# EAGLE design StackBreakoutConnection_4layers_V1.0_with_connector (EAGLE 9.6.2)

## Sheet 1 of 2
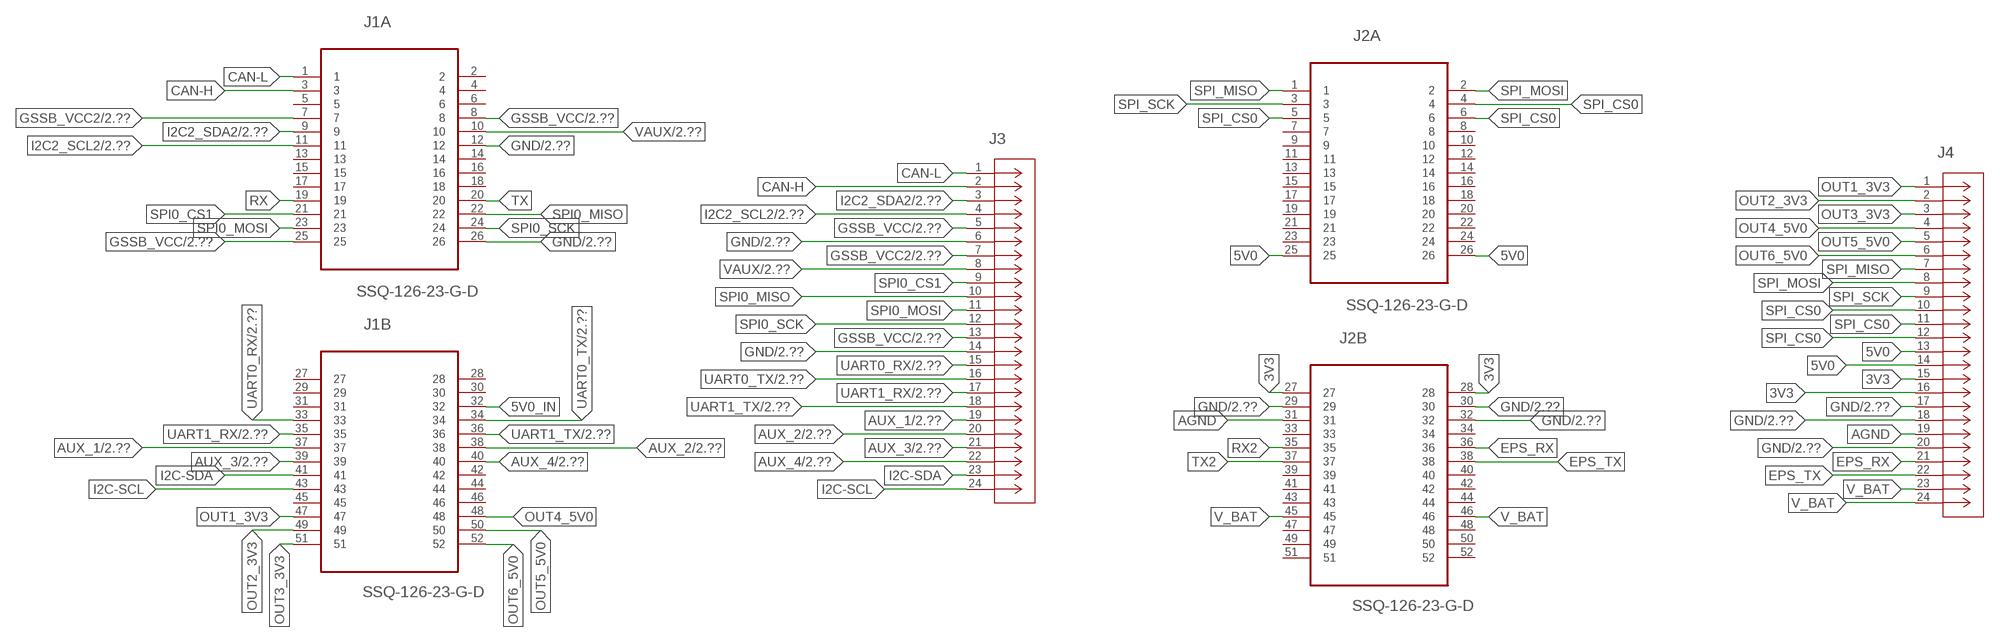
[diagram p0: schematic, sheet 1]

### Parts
J1  SSQ-126-23-G-D  [SAMTEC_SSQ-126-23-G-D]
J2  SSQ-126-23-G-D  [SAMTEC_SSQ-126-23-G-D]
J3  2086592440  [CON_2086592440_MOL]
J4  2086592440  [CON_2086592440_MOL]

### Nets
3V3: J2.27 J2.28 J4.15 J4.16
5V0: J2.25 J2.26 J4.13 J4.14
5V0_IN: J1.32
AGND: J2.31 J4.19
AUX_1: J1.37 J3.19 ; also sheet 2
AUX_2: J1.38 J3.20 ; also sheet 2
AUX_3: J1.39 J3.21 ; also sheet 2
AUX_4: J1.40 J3.22 ; also sheet 2
CAN-H: J1.3 J3.2
CAN-L: J1.1 J3.1
EPS_RX: J2.36 J4.21
EPS_TX: J2.38 J4.22
GND: J1.12 J1.26 J2.29 J2.30 J2.32 J3.6 J3.14 J4.17 J4.18 J4.20 ; also sheet 2
GSSB_VCC: J1.8 J1.25 J3.5 J3.13 ; also sheet 2
GSSB_VCC2: J1.7 J3.7 ; also sheet 2
I2C2_SCL2: J1.11 J3.4 ; also sheet 2
I2C2_SDA2: J1.9 J3.3 ; also sheet 2
I2C-SCL: J1.43 J3.24
I2C-SDA: J1.41 J3.23
OUT1_3V3: J1.47 J4.1
OUT2_3V3: J1.49 J4.2
OUT3_3V3: J1.51 J4.3
OUT4_5V0: J1.48 J4.4
OUT5_5V0: J1.50 J4.5
OUT6_5V0: J1.52 J4.6
RX: J1.19
RX2: J2.35
SPI0_CS1: J1.21 J3.9
SPI0_MISO: J1.22 J3.10
SPI0_MOSI: J1.23 J3.11
SPI0_SCK: J1.24 J3.12
SPI_CS0: J2.4 J2.5 J2.6 J4.10 J4.11 J4.12
SPI_MISO: J2.1 J4.7
SPI_MOSI: J2.2 J4.8
SPI_SCK: J2.3 J4.9
TX: J1.20
TX2: J2.37
UART0_RX: J1.33 J3.15 ; also sheet 2
UART0_TX: J1.34 J3.16 ; also sheet 2
UART1_RX: J1.35 J3.17 ; also sheet 2
UART1_TX: J1.36 J3.18 ; also sheet 2
V_BAT: J2.45 J2.46 J4.23 J4.24
VAUX: J1.10 J3.8 ; also sheet 2
Unconnected: J1.2 J1.4 J1.5 J1.6 J1.13 J1.14 J1.15 J1.16 J1.17 J1.18 J1.27 J1.28 J1.29 J1.30 J1.31 J1.42 J1.44 J1.45 J1.46 J2.7 J2.8 J2.9 J2.10 J2.11 J2.12 J2.13 J2.14 J2.15 J2.16 J2.17 J2.18 J2.19 J2.20 J2.21 J2.22 J2.23 J2.24 J2.33 J2.34 J2.39 J2.40 J2.41 J2.42 J2.43 J2.44 J2.47 J2.48 J2.49 J2.50 J2.51 J2.52

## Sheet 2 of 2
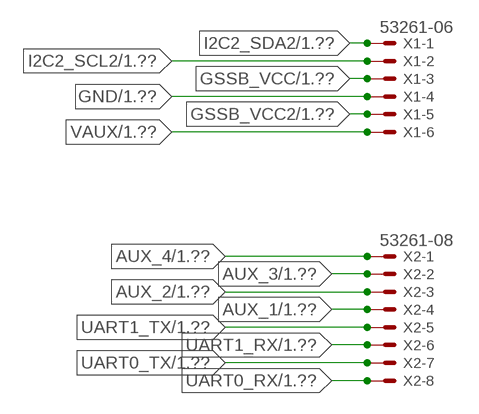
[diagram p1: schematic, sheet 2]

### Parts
X1  53261-06  [53261-06]
X2  53261-08  [53261-08]

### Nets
AUX_1: X2.4 ; also sheet 1
AUX_2: X2.3 ; also sheet 1
AUX_3: X2.2 ; also sheet 1
AUX_4: X2.1 ; also sheet 1
GND: X1.4 ; also sheet 1
GSSB_VCC: X1.3 ; also sheet 1
GSSB_VCC2: X1.5 ; also sheet 1
I2C2_SCL2: X1.2 ; also sheet 1
I2C2_SDA2: X1.1 ; also sheet 1
UART0_RX: X2.8 ; also sheet 1
UART0_TX: X2.7 ; also sheet 1
UART1_RX: X2.6 ; also sheet 1
UART1_TX: X2.5 ; also sheet 1
VAUX: X1.6 ; also sheet 1

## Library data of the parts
J1 J2 = SPEL:SSQ-126-23-G-D: CONN RECEPTACLE, 2.54MM, DUAL, 52WAY; MPN: SSQ-126-23-G-D; OC_FARNELL: -; OC_NEWARK: 82P0504; PACKAGE: RECEPTACLE, 2.54MM, DUAL, 52WAY; SUPPLIER: Samtec
J3 J4 = MolexP24:2086592440; BUILT_BY: Molex_Team; COPYRIGHT: Copyright (C) 2018 Accelerated Designs. All rights reserved; DESCRIPTION: 2.00mm Pitch, iGrid PCB Header, Dual Row, Right-Angle, Through Hole, 0.10µm Gold (Au) Plating, Positive Lock, 24 Circuits, Tray, 3.20mm PC Tail Length, Natural; MANUFACTURER_PART_NUMBER: 2086592440; SOURCELIBRARY: Add_to_database_2021-04-21; VENDOR: Molex Connector Corporation
X1 = con-molex:53?-06: CONNECTOR wire to board 1.25 mm (.049 inch) pitch header; MF: MOLEX; OC_FARNELL: 1125375; OC_NEWARK: unknown
X2 = con-molex:53?-08: CONNECTOR wire to board 1.25 mm (.049 inch) pitch header; MF: MOLEX; OC_FARNELL: 1125376; OC_NEWARK: unknown

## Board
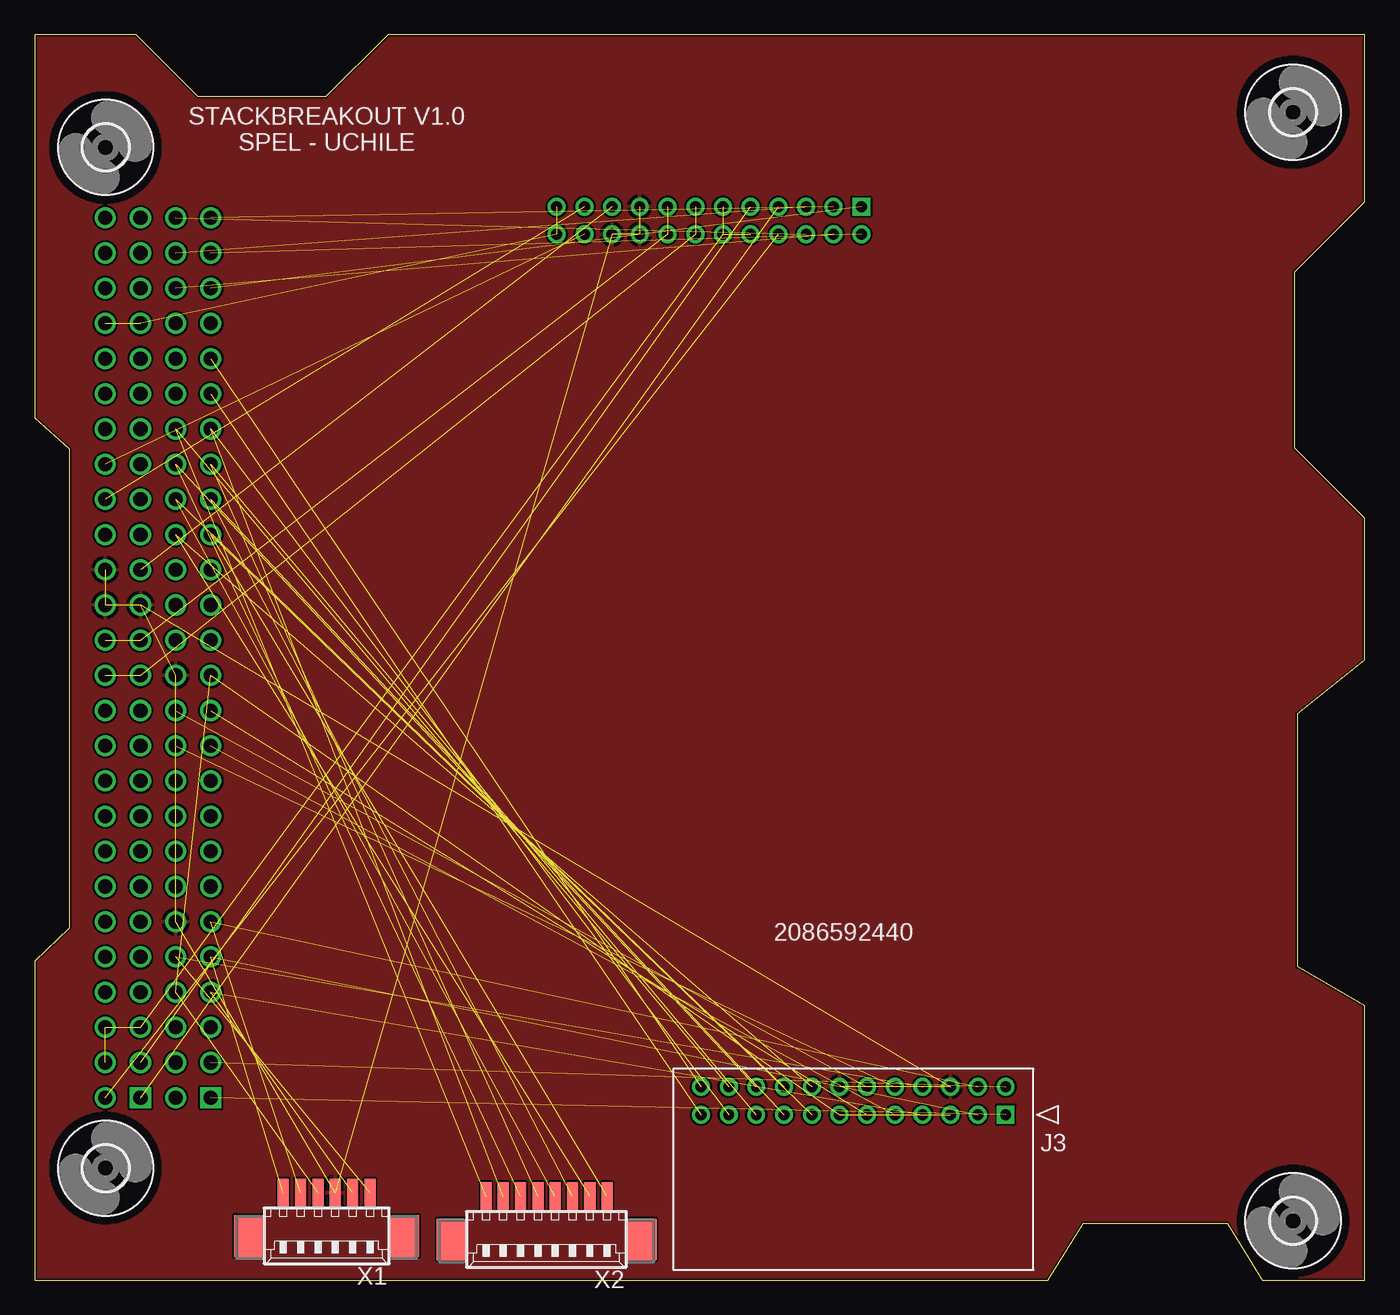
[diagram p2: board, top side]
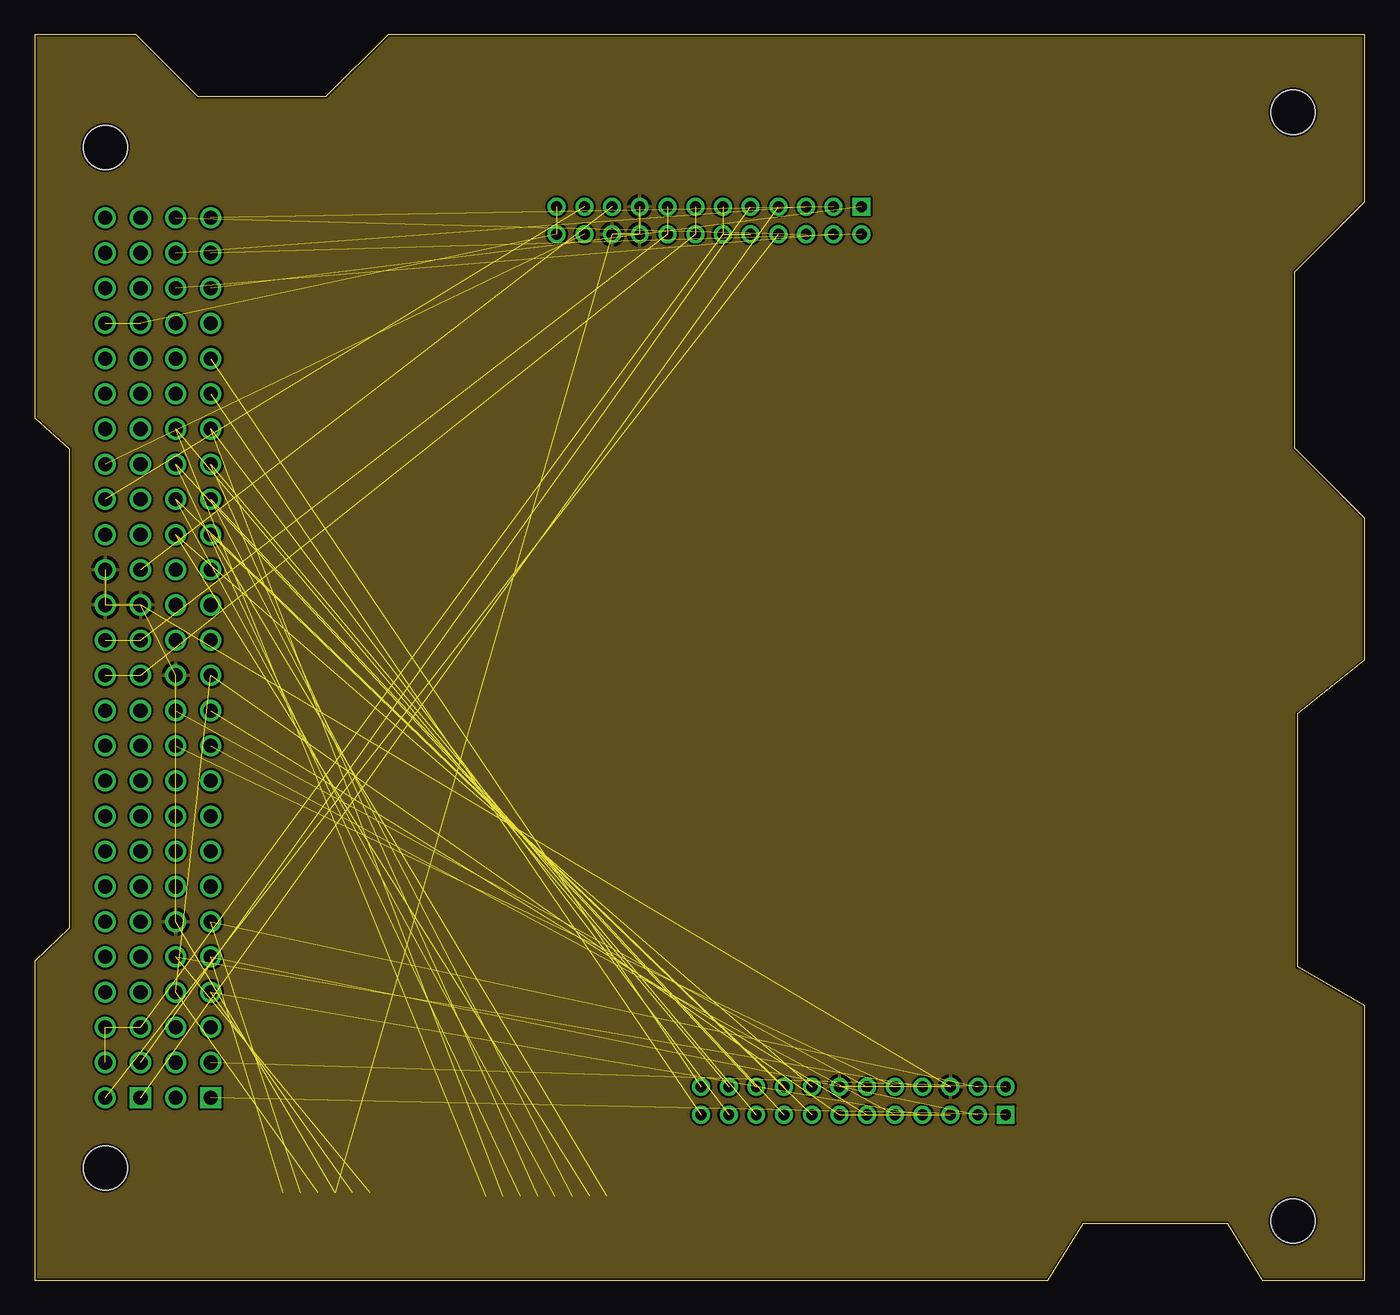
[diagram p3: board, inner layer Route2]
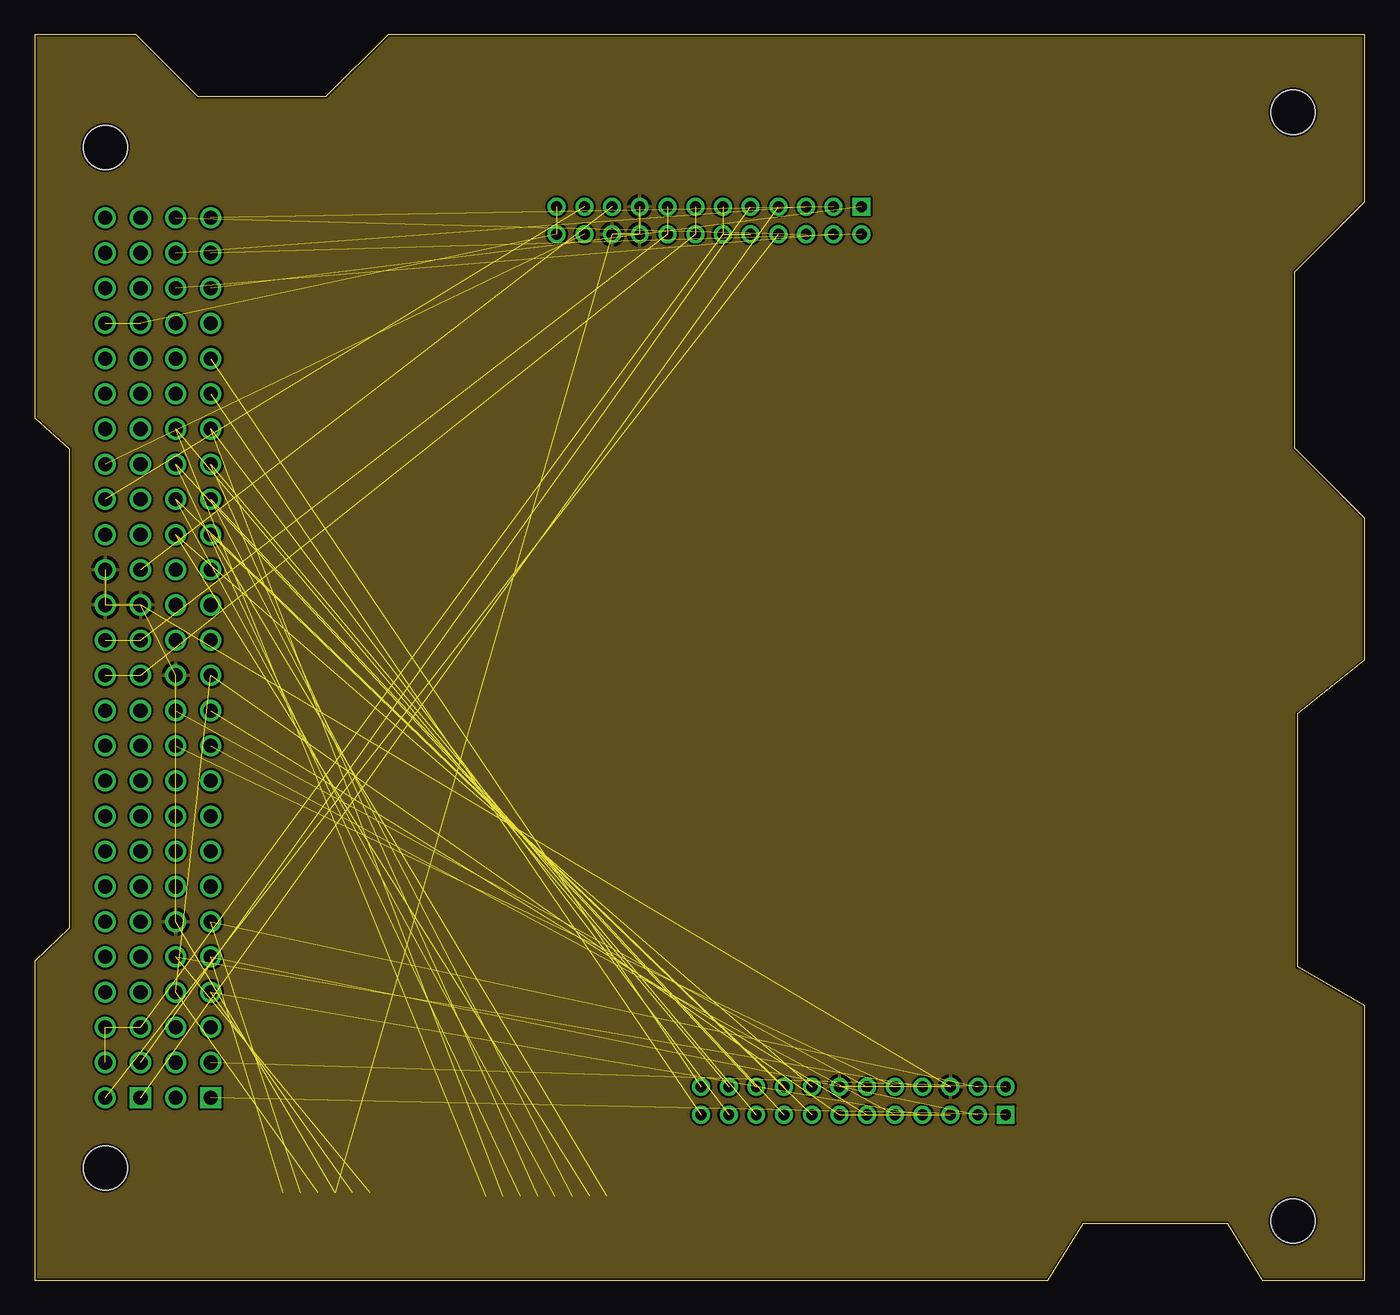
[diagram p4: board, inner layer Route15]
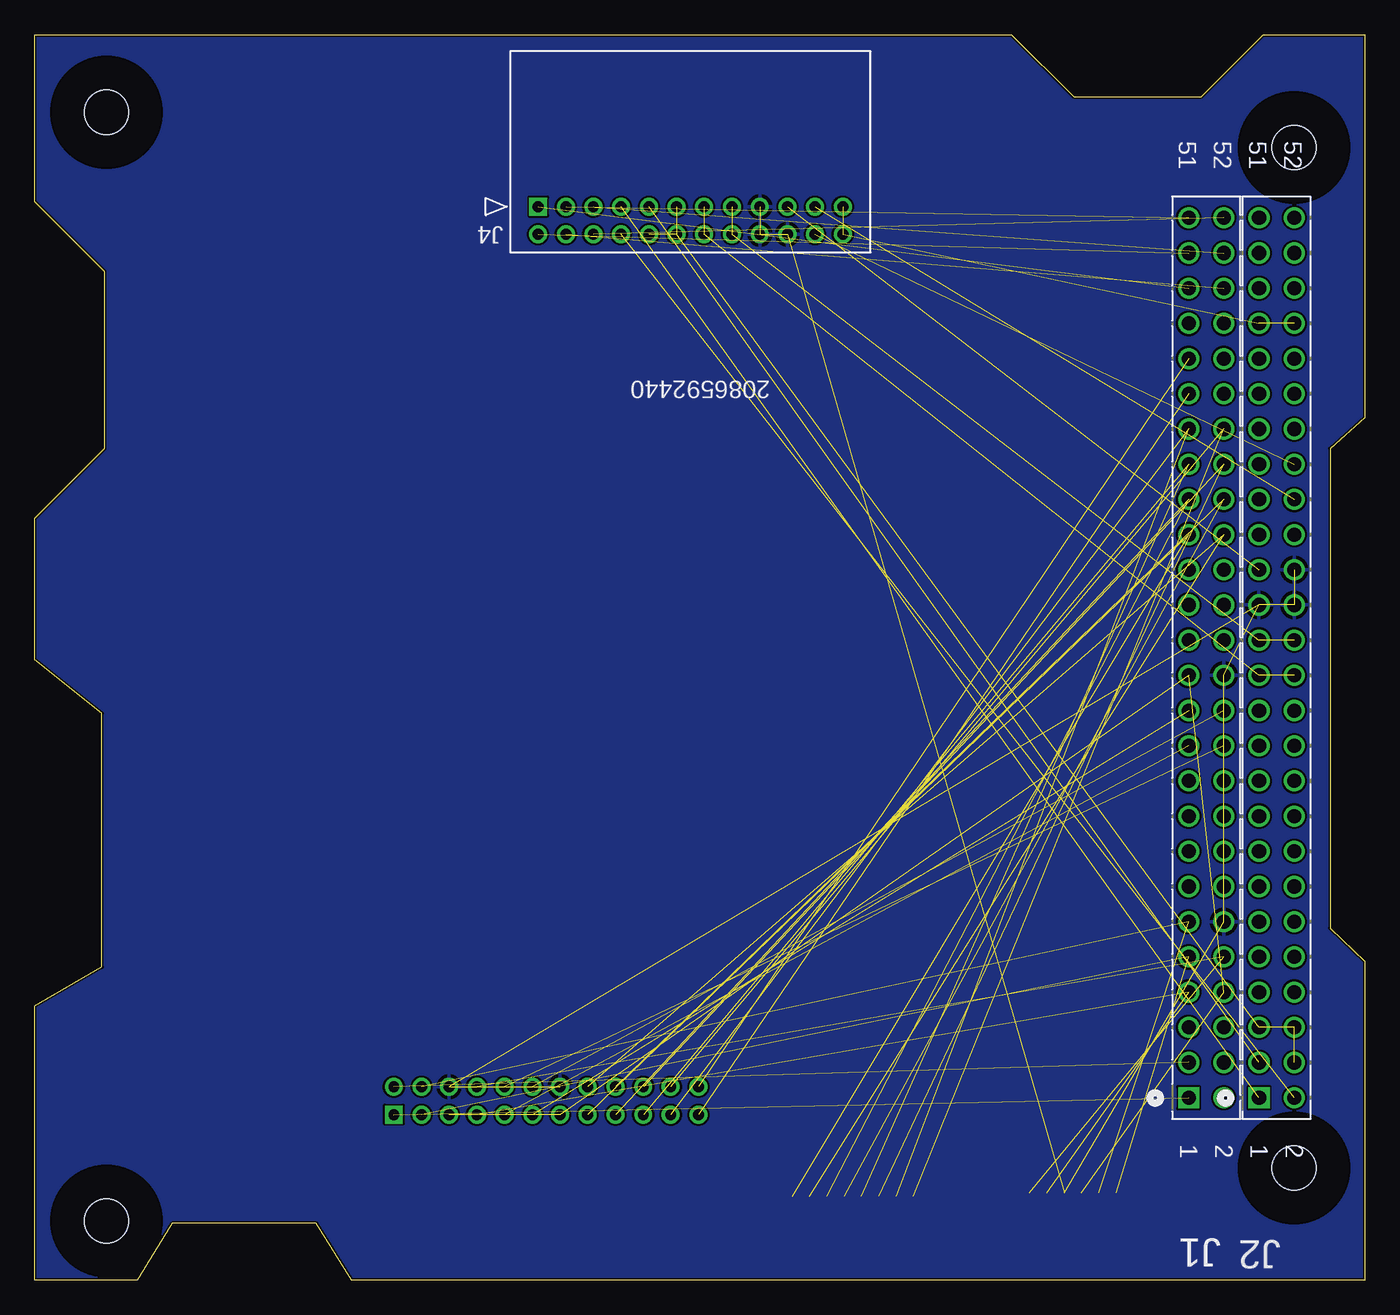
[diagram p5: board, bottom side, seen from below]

Size 96.04 x 89.88 mm. Coordinates in mm from the lower left corner, seen from the top.
Outline: 90.98,72.77 96.04,77.83 96.04,89.88 25.51,89.88 21.02,85.4 11.8,85.4 7.32,89.88 0,89.88 0,62.23 2.5,60 2.5,25.4 0,23 0,0 73.15,0 75.7,4.1 86.09,4.1 88.65,0 96.01,0 96.01,19.81 91.19,22.61 91.19,40.89 96.04,44.76 96.04,54.97 90.98,60.02 90.98,72.77
Copper layers (1+2*15+16): Top 0.035mm / dielectric 1.5mm / Route2 0.035mm / dielectric 0.15mm / Route15 0.035mm / dielectric 0.2mm / Bottom 0.035mm
Design rules "default *": minimum track width 20mil, minimum drill 0.2mm, track to track 6mil, track to pad 6mil, pad to pad 6mil, via to via 6mil, smd to smd 6mil, copper to edge 6mil, drill to drill 6mil, minimum pad ring 10mil, minimum via ring 8mil, stop-mask expansion 4mil, vias tented up to drill 0mil, thermal gap 10mil

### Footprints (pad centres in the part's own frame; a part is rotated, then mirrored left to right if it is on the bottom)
SAMTEC_SSQ-126-23-G-D = drill 1.016 square: 1 63.5,-2.54 | drill 1.016: 2 63.5,0; 3 60.96,-2.54; 4 60.96,0; 5 58.42,-2.54; 6 58.42,0; 7 55.88,-2.54; 8 55.88,0; 9 53.34,-2.54; 10 53.34,0; 11 50.8,-2.54; 12 50.8,0; 13 48.26,-2.54; 14 48.26,0; 15 45.72,-2.54; 16 45.72,0; 17 43.18,-2.54; 18 43.18,0; 19 40.64,-2.54; 20 40.64,0; 21 38.1,-2.54; 22 38.1,0; 23 35.56,-2.54; 24 35.56,0; 25 33.02,-2.54; 26 33.02,0; 27 30.48,-2.54; 28 30.48,0; 29 27.94,-2.54; 30 27.94,0; 31 25.4,-2.54; 32 25.4,0; 33 22.86,-2.54; 34 22.86,0; 35 20.32,-2.54; 36 20.32,0; 37 17.78,-2.54; 38 17.78,0; 39 15.24,-2.54; 40 15.24,0; 41 12.7,-2.54; 42 12.7,0; 43 10.16,-2.54; 44 10.16,0; 45 7.62,-2.54; 46 7.62,0; 47 5.08,-2.54; 48 5.08,0; 49 2.54,-2.54; 50 2.54,0; 51 0,-2.54; 52 0,0
CON_2086592440_MOL = drill 0.787 pad 1.143 square: 1 0,0 | drill 0.787 pad 1.143: 2 0,2.007; 3 -2.007,0; 4 -2.007,2.007; 5 -3.988,0; 6 -3.988,2.007; 7 -5.994,0; 8 -5.994,2.007; 9 -8.001,0; 10 -8.001,2.007; 11 -10.008,0; 12 -10.008,2.007; 13 -11.989,0; 14 -11.989,2.007; 15 -13.995,0; 16 -13.995,2.007; 17 -16.002,0; 18 -16.002,2.007; 19 -18.009,0; 20 -18.009,2.007; 21 -19.99,0; 22 -19.99,2.007; 23 -21.996,0; 24 -21.996,2.007
3,2 = hole 3.2: 0,0
53261-06 = smd 0.8 x 2: 1 3.125,-2.5; 2 1.875,-2.5; 3 0.625,-2.5; 4 -0.625,-2.5; 5 -1.875,-2.5; 6 -3.125,-2.5 | smd 2.1 x 3: S1 5.625,0.625; S2 -5.625,0.625
53261-08 = smd 0.8 x 2: 1 4.375,-2.5; 2 3.125,-2.5; 3 1.875,-2.5; 4 0.625,-2.5; 5 -0.625,-2.5; 6 -1.875,-2.5; 7 -3.125,-2.5; 8 -4.375,-2.5 | smd 2.1 x 3: S1 6.875,0.625; S2 -6.875,0.625

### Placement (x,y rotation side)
J1  10.18,76.66 270 bottom
J2  5.1,76.66 270 bottom
J3  70.1,11.94 0 top
J4  59.69,77.47 180 bottom
U$1  [3,2]  5.12,81.74 0 top
U$2  [3,2]  90.85,84.28 0 top
U$3  [3,2]  90.85,4.27 0 top
U$4  [3,2]  5.12,8.08 0 top
X1  21.08,3.81 180 top
X2  36.96,3.56 180 top

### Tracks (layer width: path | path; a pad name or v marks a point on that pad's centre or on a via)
3V3  (3 unrouted)
5V0  (3 unrouted)
AGND  (1 unrouted)
AUX_1  (2 unrouted)
AUX_2  (2 unrouted)
AUX_3  (2 unrouted)
AUX_4  (2 unrouted)
CAN-H  (1 unrouted)
CAN-L  (1 unrouted)
EPS_RX  (1 unrouted)
EPS_TX  (1 unrouted)
GND  (10 unrouted)
  pour Route15: -0.22,90.12 7.77,90.12 7.77,90.04 12.04,85.77 20.96,85.77 26.02,90.83 96.4,90.83 96.71,90.52 96.71,77.77 91.45,72.52 91.45,60.39 96.5,55.34 96.5,44.84 91.56,39.9 91.56,22.84 96.45,20.03 96.45,-0.36 88.28,-0.36 85.72,3.61 76.26,3.61 73.9,-0.36 -0.35,-0.36 -0.35,23.1 2.23,25.67 2.23,59.72 -0.23,62.18 -0.23,90.12 -0.23,90.12
  pour Top: -0.25,-0.13 73.41,-0.13 76.03,3.81 85.89,3.81 88.6,-0.25 96.27,-0.25 96.27,20.57 91.44,22.99 91.44,40.58 96.27,44.2 96.27,55.24 91.31,60.2 91.31,72.64 96.39,77.72 96.39,90.17 24.89,90.17 20.57,85.85 11.65,85.85 8.22,90.42 -0.25,90.42 -0.25,62.23 2.29,59.69 2.29,25.65 -0.25,23.11
  pour Route2: -0.46,-0.28 73.46,-0.28 76.08,3.66 85.9,3.66 88.53,-0.28 96.32,-0.28 96.32,20.42 91.87,22.64 91.87,40.87 96.32,44.2 96.32,55.22 91.36,60.17 91.36,72.62 96.44,77.7 96.44,90.4 25.32,90.4 20.75,85.83 11.77,85.83 8.62,90.02 -0.2,90.02 -0.2,62.33 2.08,60.05 2.08,25.88 -0.46,23.34
  pour Bottom: -0.27,90.34 7.08,90.34 7.08,90.4 11.74,85.74 11.74,85.86 20.77,85.86 26.09,91.18 95.59,91.18 96.65,90.11 96.65,77.24 91.53,72.11 91.53,60.11 96.71,54.93 96.71,44.56 91.64,39.49 91.64,22.93 96.27,20.25 96.27,-0.51 88.48,-0.51 85.92,3.45 76.54,3.45 74.18,-0.51 -0.4,-0.51 -0.4,23.33 2.18,25.9 2.18,59.57 -0.28,62.03 -0.28,90.35 -0.28,90.35
GSSB_VCC  (4 unrouted)
GSSB_VCC2  (2 unrouted)
I2C2_SCL2  (2 unrouted)
I2C2_SDA2  (2 unrouted)
I2C-SCL  (1 unrouted)
I2C-SDA  (1 unrouted)
OUT1_3V3  (1 unrouted)
OUT2_3V3  (1 unrouted)
OUT3_3V3  (1 unrouted)
OUT4_5V0  (1 unrouted)
OUT5_5V0  (1 unrouted)
OUT6_5V0  (1 unrouted)
SPI0_CS1  (1 unrouted)
SPI0_MISO  (1 unrouted)
SPI0_MOSI  (1 unrouted)
SPI0_SCK  (1 unrouted)
SPI_CS0  (5 unrouted)
SPI_MISO  (1 unrouted)
SPI_MOSI  (1 unrouted)
SPI_SCK  (1 unrouted)
UART0_RX  (2 unrouted)
UART0_TX  (2 unrouted)
UART1_RX  (2 unrouted)
UART1_TX  (2 unrouted)
V_BAT  (3 unrouted)
VAUX  (2 unrouted)

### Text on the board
tPlace: STACKBREAKOUT V1.0 / SPEL - UCHILE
